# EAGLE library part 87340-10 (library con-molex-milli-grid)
RECEPTACAL
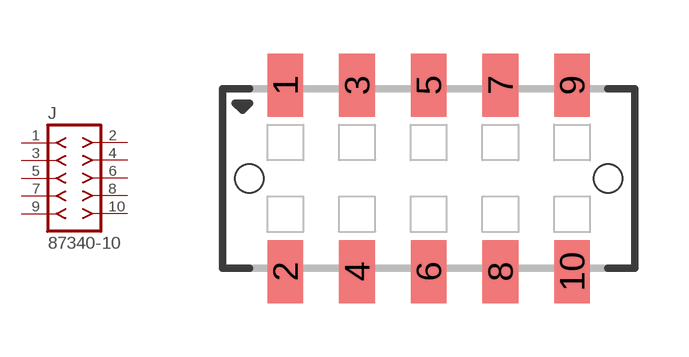
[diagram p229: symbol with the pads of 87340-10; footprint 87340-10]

Designator prefix J

## 87340-10  [87340-10]
1  1  pas
2  2  pas
3  3  pas
4  4  pas
5  5  pas
6  6  pas
7  7  pas
8  8  pas
9  9  pas
10  10  pas

## Footprint 87340-10 (pad centres in mm)
RECEPTACAL SMD Dual Row, Vertical, Low Profile
smd 1 x 1.75: 1 -4,2.6; 2 -4,-2.6; 3 -2,2.6; 4 -2,-2.6; 5 0,2.6; 6 0,-2.6; 7 2,2.6; 8 2,-2.6; 9 4,2.6; 10 4,-2.6
hole 0.8 at -5,0
hole 0.8 at 5,0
